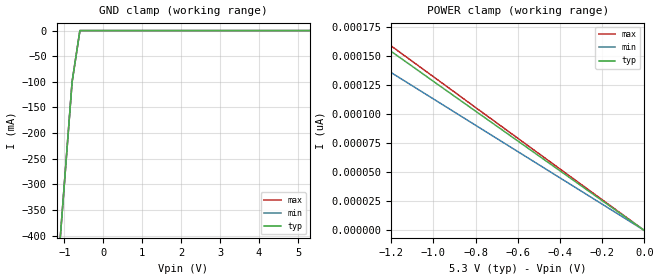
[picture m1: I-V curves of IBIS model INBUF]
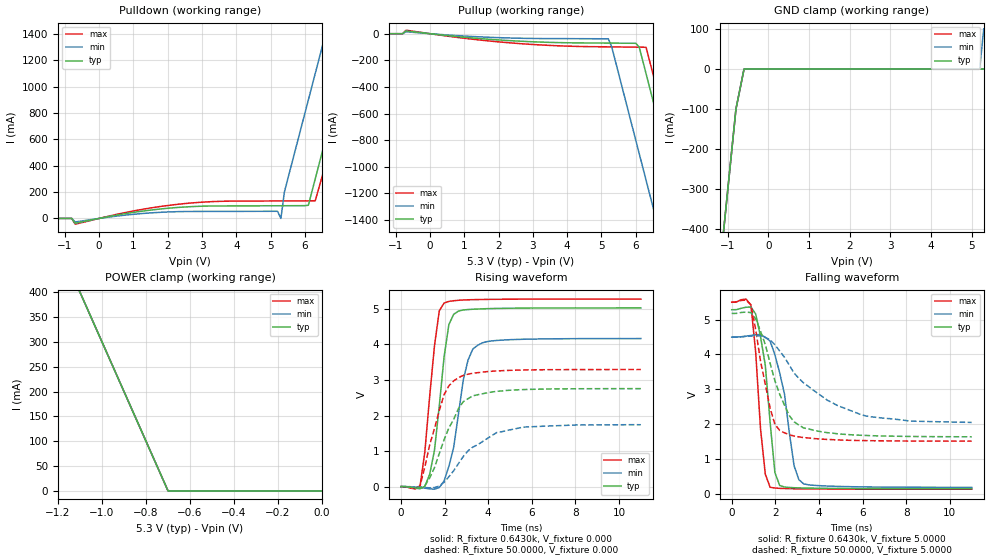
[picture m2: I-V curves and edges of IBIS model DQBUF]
| IBIS file m48z58y.ibs created by s2ibis2 version 1.1
| North Carolina State University Electronics Research Laboratory  1995
[IBIS ver]   2.1
[File name]   m48z58y.ibs
[File Rev]   3.0
[Date]   December 9, 2005
[Source]   ST models
[Notes]   Extracted view used. Simulation with Eldo (the s2ibis2 code
   was slightly changed to run with Eldo)
[Disclaimer] We used the packaging information of the T212. It should be
   the same but need to be confirme. We also put a 1.0 ohm
   resistor in series with the output and input for current
   limitation.
[Copyright]   ST Microelectronics Inc.
|   Component m48t58y
[Component]   m48t58y
[Manufacturer]   ST Microelectronics [Package]
[Package]
| variable   typ   min   max
R_pkg   55.0000m   45.0000m   65.0000m
L_pkg   6.7000nH   4.2000nH   9.2000nH
C_pkg   1.1000pF   0.6000pF   1.6000pF
[Pin]  signal_name   model_name   R_pin   L_pin   C_pin
| gdb  dummy   dummy
| od   dummy   dummy
1   NC   NC
2   A12   INBUF
3   A7   INBUF
4   A6   INBUF
5   A5   INBUF
6   A4   INBUF
7   A3   INBUF
8   A2   INBUF
9   A1   INBUF
10   A0   INBUF
11   DQ0   DQBUF
12   DQ1   DQBUF
13   DQ2   DQBUF
14   VSS   GND
15   DQ3   DQBUF
16   DQ4   DQBUF
17   DQ5   DQBUF
18   DQ6   DQBUF
19   DQ7   DQBUF
20   E#   INBUF
21   A10   INBUF
22   G#   INBUF
23   A11   INBUF
24   A9   INBUF
25   A8   INBUF
26   NC   NC
27   W#   INBUF
28   VCC   POWER
| Models and submodels in the file (2): INBUF (Input), DQBUF (I/O)
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|   Model INBUF
[Model]   INBUF
Model_type   Input
Vinl =   0.8000V
Vinh =   2.2000V
C_comp   2.0100pF   1.9700pF   2.0600pF
[Temperature Range]   27.0000   70.0000   0.000
[Voltage Range]   5.3000V   4.5000V   5.5000V
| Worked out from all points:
|   GND clamp passes 1 mA (typ) near -0.60 V on its own axis
[GND_clamp]
| voltage   I(typ)   I(min)   I(max)
-5V       -4.3A      -4.3A      -4.3A
-1.2V     -500mA     -500mA     -500mA
-1V       -300mA     -300mA     -300mA
-800mV    -100mA     -100mA     -100mA
-600mV    -2.424uA   -939.7nA   -1.758uA
5.3V      12.61pA    12.7pA     12.61pA
[POWER_clamp]
| voltage   I(typ)   I(min)   I(max)
-5V       640.7pA    564.8pA    660.3pA
-1.6V     205pA      180.7pA    211.3pA
-1.5V     192.2pA    169.4pA    198.1pA
-1.4V     179.4pA    158.1pA    184.9pA
-1.3V     166.6pA    146.9pA    171.7pA
0V        0A         0A         0A
|   Model DQBUF
[Model]   DQBUF
Model_type   I/O
Polarity   Inverting
Enable   Active-High
Vinl =   0.8000V
Vinh =   2.2000V
Vmeas =   1.5000V
Cref =1.000e-10F
Rref =   0.6430k
Vref =   1.7500V
C_comp   4.3700pF   4.2600pF   4.4800pF
[Temperature Range]   27.0000   70.0000   0.000
[Voltage Range]   5.3000V   4.5000V   5.5000V
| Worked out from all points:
|   slope of the pulldown table from 0 to 0.795 V, typ, clamps not added: 21.1 ohm
|   slope of the pullup table from 0 to 0.795 V, typ, clamps not added: 36.8 ohm
|   GND clamp passes 1 mA (typ) near -0.60 V on its own axis
|   POWER clamp passes 1 mA (typ) near -0.70 V on its own axis
|   rising waveform, R_fixture 0.6430k, V_fixture 0.000: 20-80 % time 536ps typ, 681ps min, 489ps max; typ from 0 V to 5.03 V
|   rising waveform, R_fixture 50.0000, V_fixture 0.000: 20-80 % time 1.1ns typ, 1.77ns min, 888ps max; typ from 0 V to 2.76 V
|   falling waveform, R_fixture 0.6430k, V_fixture 5.0000: 20-80 % time 505ps typ, 674ps min, 392ps max; typ from 5.29 V to 0.146 V
|   falling waveform, R_fixture 50.0000, V_fixture 5.0000: 20-80 % time 1.13ns typ, 2.52ns min, 728ps max; typ from 5.18 V to 1.64 V
[Pulldown]
| voltage   I(typ)   I(min)   I(max)
-5V       0A         0A         0A
-700mV    -36.61mA   -26.81mA   -43.63mA
2.4V      85.18mA    51.98mA    110.1mA
5.2V      96.11mA    54.24mA    132.6mA
5.3V      96.2mA     0A         132.7mA
5.4V      96.29mA    200mA      132.8mA
6.1V      100mA      900mA      133.5mA
6.3V      300mA      1.1A       133.8mA
6.7V      700mA      1.5A       500mA
7.5V      1.5A       2.3A       1.3A
7.9V      1.9A       2.7A       1.7A
10.3V     4.3A       5.1A       4.1A
[Pullup]
| voltage   I(typ)   I(min)   I(max)
-5V       0A         0A         0A
-700mV    20.85mA    14.65mA    26.3mA
5.2V      -70.61mA   -38.29mA   -98.8mA
5.3V      -70.79mA   -100mA     -99.08mA
6V        -72.11mA   -800mA     -101mA
6.1V      -100mA     -900mA     -101.3mA
6.3V      -300mA     -1.1A      -102.1mA
6.7V      -700mA     -1.5A      -500mA
7.1V      -1.1A      -1.9A      -900mA
7.5V      -1.5A      -2.3A      -1.3A
7.9V      -1.9A      -2.7A      -1.7A
10.3V     -4.3A      -5.1A      -4.1A
[GND_clamp]
| voltage   I(typ)   I(min)   I(max)
-5V       -4.3A      -4.3A      -4.3A
-1.2V     -500mA     -500mA     -500mA
-1V       -300mA     -300mA     -300mA
-800mV    -100mA     -100mA     -100mA
-600mV    -26.04uA   -10.29uA   -17.63uA
5.2V      -9.602nA   2.467uA    43.19pA
5.3V      -46.34pA   100mA      43.03pA
[POWER_clamp]
| voltage   I(typ)   I(min)   I(max)
-5V       4.3A       4.3A       4.3A
-1.1V     400mA      400mA      400mA
-1V       300mA      300mA      300mA
-700mV    12.45uA    2.467uA    49.04uA
0V        0A         0A         0A
[Ramp]
| variable   typ   min   max
dV/dt_r   3.0170/0.5109n   2.5001/0.7604n   3.1666/0.3988n
dV/dt_f   3.0873/0.4480n   2.5897/0.7615n   3.2207/0.3285n
R_load = 0.6430k
[Rising Waveform]
R_fixture = 0.6430k
V_fixture = 0.000
V_fixture_min = 0.000
V_fixture_max = 0.000
| time   V(typ)   V(min)   V(max)
0s        1.106nV    1.375nV    928.6pV
880ps     -60.33mV   -22.31mV   11.99mV
1.1ns     9.409mV    -43.89mV   984.9mV
1.54ns    1.022V     -71.76mV   3.96V
1.76ns    2.266V     -27.2mV    4.945V
1.98ns    3.647V     159.3mV    5.164V
2.42ns    4.848V     1.104V     5.231V
2.86ns    4.971V     3.005V     5.252V
3.52ns    4.997V     3.975V     5.263V
11ns      5.028V     4.167V     5.278V
[Rising Waveform]
R_fixture = 50.0000
V_fixture = 0.000
V_fixture_min = 0.000
V_fixture_max = 0.000
| time   V(typ)   V(min)   V(max)
0s        826.7pV    937.9pV    728pV
880ps     -40.65mV   -16.02mV   23.78mV
1.32ns    242.2mV    -33.18mV   1.174V
1.98ns    1.318V     120.7mV    2.585V
2.2ns     1.652V     278.6mV    2.836V
2.64ns    2.195V     648.5mV    3.067V
3.3ns     2.555V     1.113V     3.19V
4.4ns     2.682V     1.523V     3.256V
5.72ns    2.733V     1.678V     3.283V
11ns      2.757V     1.742V     3.295V
[Falling Waveform]
R_fixture = 0.6430k
V_fixture = 5.0000
V_fixture_min = 4.5000
V_fixture_max = 5.5000
| time   V(typ)   V(min)   V(max)
0s        5.285V     4.5V       5.5V
880ps     5.362V     4.545V     5.421V
1.1ns     5.162V     4.568V     4.057V
1.54ns    3.691V     4.494V     562.2mV
1.76ns    2.05V      4.386V     187.5mV
1.98ns    608.4mV    3.991V     164.3mV
2.2ns     236.8mV    3.47V      155.5mV
2.86ns    173.4mV    800.6mV    143.4mV
3.3ns     165.4mV    283.7mV    140.3mV
11ns      145.6mV    183.9mV    132.1mV
[Falling Waveform]
R_fixture = 50.0000
V_fixture = 5.0000
V_fixture_min = 4.5000
V_fixture_max = 5.5000
| time   V(typ)   V(min)   V(max)
0s        5.178V     4.5V       5.5V
880ps     5.204V     4.529V     5.429V
1.32ns    4.671V     4.535V     3.813V
1.76ns    3.751V     4.422V     2.46V
1.98ns    3.245V     4.278V     1.994V
2.2ns     2.857V     4.099V     1.818V
2.64ns    2.245V     3.692V     1.695V
3.3ns     1.889V     3.181V     1.614V
5.94ns    1.679V     2.269V     1.528V
11ns      1.636V     2.05V      1.511V
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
